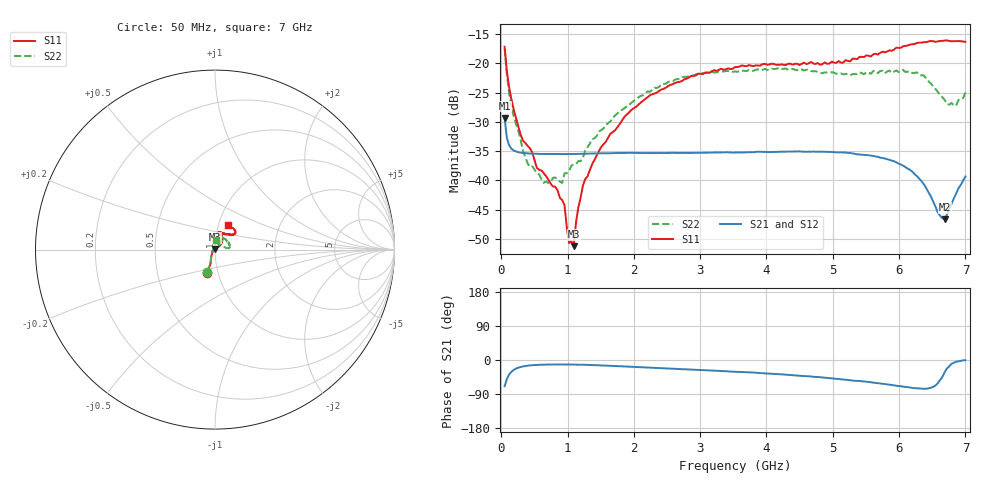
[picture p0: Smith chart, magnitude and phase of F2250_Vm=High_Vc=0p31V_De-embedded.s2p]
! Integrated Device Technology
! Corporate Headquarters
! 6024 Silver Creek Valley Road
! San Jose, CA 95138  USA
! Phone:  1-408-284-8200
! Toll Free:  1-800-223-1366
! Webpage:  http://www.idt.com/
! Timing and RF Division
! 515 Groton Road, Suite 102
! Westford, MA 01886-6024
! Device:  F2250
! Description: Voltage Variable RF Attenuator
! Frequency:  50.0 -  6000.00 MHz
! Package:  3x3 mm Thin QFN Plastic Package: 16 pin
! Ports:  2 RF, 3 DC
!  Pin  1  = GND
!  Pin  2  = NC
!  Pin  3  = RF1  = Port 1
!  Pin  4  = NC
!  Pin  5  = GND
!  Pin  6  = GND
!  Pin  7  = GND
!  Pin  8  = GND
!  Pin  9  = NC
!  Pin 10  = RF2  = Port 2
!  Pin 11  = NC
!  Pin 12  = GND
!  Pin 13  = GND
!  Pin 14  = VCNTRL
!  Pin 15  = VDD
!  Pin 16  = VMODE
! Vcntrl:  0.310 Volts
! Vmode:  +3.300 Volts
! Vdd:  +3.30  Volts
! Current:  1.253 mA
! Data:  The device was measured on a the F2250 evaluation board which has
!  individual transmission lines to the RF pins.  Data was collected
!  using a calibrated network analyzer.  The evaluation board was
!  de-embedded using a TRL calibration technique.
!  The reference plane is the edge of the package pin.
! Misc:  SN 10
!  Action Tracker AT0258
! Date Measured:  2014-11-26
! Date:  2015-10-15  MJV
! Note:
!  Integrated Device Technology supplies this data as a sample of measured
!  data at the package pin for this product.  Your particular data for this
!  product may vary.
!  Data was taken at 25 degrees C.
!  Integrated Device Technology reserves the right to change this data at anytime.
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# GHz S dB R 50
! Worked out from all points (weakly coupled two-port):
!   201 points, 50 MHz to 7 GHz, reference 50 ohm
!   highest |S21| = -29.36 dB at 50 MHz (marker M1); lowest = -46.7 dB at 6.687 GHz (marker M2)
!   lowest |S11| = -51.3 dB at 1.093 GHz (marker M3), VSWR 1.01, Z = 50 + j0.273 ohm
!   |S11| at or under -10 dB: start of sweep to end of sweep
!   |S22| runs from -40.5 to -17.5 dB; largest |S21 - S12| = 5.5e-05
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0.05  -17.18 -108.5  -29.36 -69.2  -29.36 -69.2  -17.46 -110.1
0.08475  -21.46 -107.4  -32.81 -49.8  -32.82 -49.8  -22.01 -108.0
0.189  -28.00 -120.0  -34.92 -26.0  -34.92 -26.0  -29.10 -122.1
0.29325  -32.28 -127.4  -35.28 -18.4  -35.29 -18.4  -33.19 -129.9
0.3975  -34.12 -142.1  -35.41 -15.0  -35.41 -15.0  -37.12 -155.2
0.5365  -37.90 -154.6  -35.48 -12.9  -35.48 -12.9  -38.86 -178.7
0.64075  -38.80 -162.7  -35.51 -12.2  -35.51 -12.2  -40.44 158.5
0.91875  -43.39 156.2  -35.53 -11.8  -35.53 -11.8  -40.46 120.8
0.9535  -44.24 171.2  -35.53 -11.8  -35.53 -11.8  -38.82 117.9
1.023  -50.74 140.6  -35.52 -11.9  -35.52 -11.9  -38.41 100.5
1.0925  -51.27 88.9  -35.51 -12.1  -35.50 -12.1  -37.31 91.2
1.12725  -47.20 61.4  -35.50 -12.2  -35.49 -12.2  -37.24 84.0
1.2315  -40.88 40.7  -35.46 -12.5  -35.46 -12.5  -36.12 70.1
1.6485  -32.03 41.2  -35.38 -15.3  -35.38 -15.3  -29.89 56.6
2.37825  -24.76 46.7  -35.33 -21.2  -35.33 -21.2  -24.05 52.2
3.525  -20.66 71.7  -35.26 -30.8  -35.26 -30.8  -21.40 72.1
4.7065  -20.06 72.0  -35.10 -44.1  -35.10 -44.2  -21.38 69.8
5.85325  -17.79 40.6  -36.52 -65.0  -36.52 -65.2  -21.25 22.5
6.3745  -16.40 41.0  -40.68 -76.0  -40.69 -76.0  -22.08 6.4
6.68725  -16.11 47.9  -46.67 -32.4  -46.64 -32.0  -26.25 27.7
6.861  -16.21 54.5  -42.28 -4.7  -42.26 -4.8  -27.24 57.6
7  -16.32 62.4  -39.35 -0.9  -39.32 -1.0  -24.99 84.3
